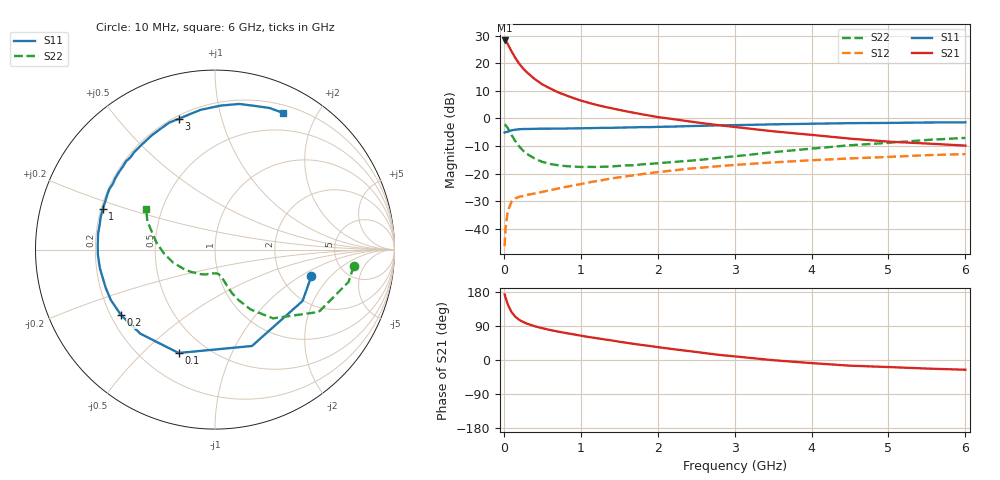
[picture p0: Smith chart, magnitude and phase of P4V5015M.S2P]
! SIEMENS Small Signal Semiconductors
! BFP182
! Si NPN RF Bipolar Junction Transistor in SOT143
! VCE = 0.5 V  IC = 15 mA
! Common Emitter S-Parameters:  March  1996
# GHz  S  MA  R  50
!  f  S11  S21  S12  S22
! GHz  MAG  ANG  MAG  ANG  MAG  ANG  MAG  ANG
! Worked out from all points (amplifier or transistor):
!   36 points, 10 MHz to 6 GHz, reference 50 ohm
!   highest |S21| = 28.2 dB at 10 MHz (marker M1)
!   |S21| within 3 dB of that: start of sweep to 82.39 MHz
!   unconditionally stable (mu >= 1): start of sweep to 11.32 MHz; 310.6 MHz to end of sweep
!   at 250 MHz: K = 0.85, MSG = 23.1 dB, |S12| = -28.0 dB
!   at 1.4 GHz: K = 2.11, MAG = 6.7 dB, |S12| = -21.7 dB
!   at 6 GHz: K = 1.76, MAG = -3.5 dB, |S12| = -12.9 dB
!   S11 on the Smith chart (normalised r, x): 10 MHz: 2.91, -1.26; 100 MHz: 0.35, -0.65; 200 MHz: 0.24, -0.30; 1 GHz: 0.21, +0.17; 3 GHz: 0.22, +0.74; 6 GHz: 0.29, +1.58
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0.01  0.5568 -15.6  25.76 172.9  0.0049 78.5  0.7786 -6.8
0.02  0.5656 -30.4  25.4 166.2  0.0097 74.7  0.765 -13.7
0.05  0.5752 -69.0  22.31 147.2  0.021 61.9  0.6744 -31.0
0.1  0.6107 -109.4  16.34 126.4  0.0312 43.7  0.5014 -49.8
0.15  0.6265 -131.6  12.42 114.1  0.0358 37.3  0.3876 -59.3
0.2  0.6383 -145.2  9.786 106.0  0.0383 34.0  0.3122 -64.8
0.25  0.6447 -154.2  8.014 100.3  0.0396 32.4  0.2619 -68.6
0.3  0.6451 -160.8  6.812 96.1  0.0414 32.8  0.2287 -70.4
0.4  0.6497 -170.7  5.178 89.1  0.044 33.7  0.1888 -73.3
0.5  0.6534 -177.6  4.139 84.0  0.047 35.1  0.1639 -75.9
0.6  0.6541 177.2  3.501 79.2  0.0503 37.3  0.1506 -78.1
0.7  0.6572 172.2  2.995 75.2  0.0539 39.0  0.1427 -80.1
0.8  0.6573 167.9  2.645 71.4  0.0576 40.1  0.1378 -82.1
1  0.6647 160.1  2.109 64.2  0.065 42.2  0.1326 -87.2
1.1  0.6676 156.5  1.925 60.8  0.0696 42.6  0.1331 -90.8
1.6  0.6875 141.0  1.34 45.3  0.0903 42.6  0.1417 -104.6
2.2  0.7133 124.8  0.973 28.7  0.1148 39.2  0.163 -123.4
3  0.7563 105.5  0.702 9.6  0.1444 32.2  0.2066 -149.2
3.5  0.7826 96.0  0.586 -0.5  0.1605 27.3  0.2456 -163.2
4.5  0.8228 80.5  0.432 -15.0  0.1892 17.8  0.3278 173.4
5.5  0.8454 68.9  0.352 -22.6  0.2168 8.6  0.4085 157.3
6  0.8508 63.6  0.323 -25.7  0.2268 3.3  0.4451 149.5
